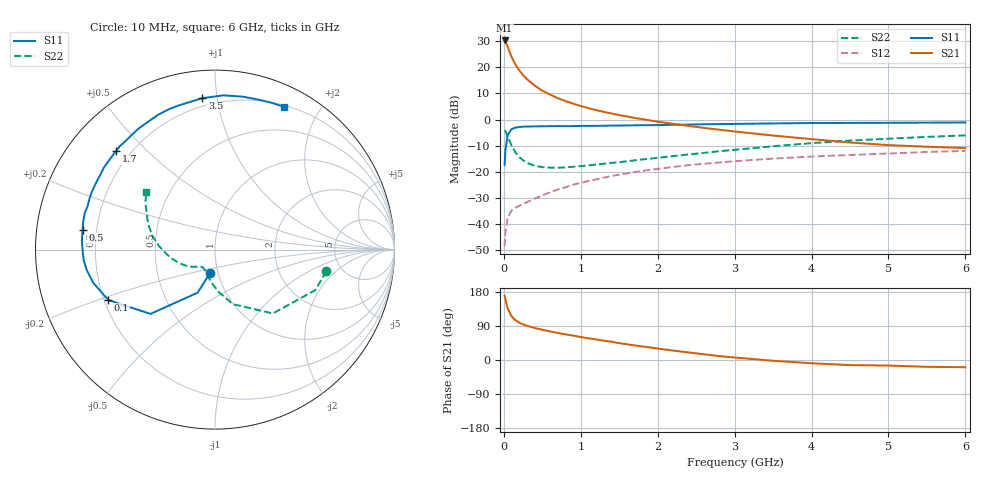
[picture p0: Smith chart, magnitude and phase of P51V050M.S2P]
! SIEMENS Small Signal Semiconductors
! BFP183
! Si NPN RF Bipolar Junction Transistor in SOT143
! VCE = 1 V  IC = 50 mA
! Common Emitter S-Parameters:  March  1996
# GHz  S  MA  R  50
!  f  S11  S21  S12  S22
! GHz  MAG  ANG  MAG  ANG  MAG  ANG  MAG  ANG
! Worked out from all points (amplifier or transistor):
!   36 points, 10 MHz to 6 GHz, reference 50 ohm
!   highest |S21| = 30.3 dB at 10 MHz (marker M1)
!   |S21| within 3 dB of that: start of sweep to 57.36 MHz
!   unconditionally stable (mu >= 1): start of sweep to 34.36 MHz; 150 MHz to end of sweep
!   at 250 MHz: K = 1.32, MAG = 21.3 dB, |S12| = -32.3 dB
!   at 1.4 GHz: K = 1.90, MAG = 6.5 dB, |S12| = -21.6 dB
!   at 6 GHz: K = 1.53, MAG = -3.7 dB, |S12| = -12.0 dB
!   S11 on the Smith chart (normalised r, x): 10 MHz: 0.91, -0.25; 100 MHz: 0.22, -0.21; 500 MHz: 0.15, +0.07; 1.7 GHz: 0.15, +0.40; 3.5 GHz: 0.15, +0.91; 6 GHz: 0.22, +1.57
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0.01  0.1361 -102.5  32.69 169.6  0.0038 64.0  0.6319 -11.0
0.02  0.2584 -111.9  31.52 159.5  0.0069 64.8  0.6033 -21.9
0.05  0.5075 -135.1  24.7 135.9  0.0133 53.1  0.4802 -47.8
0.1  0.6576 -154.7  15.89 115.5  0.0183 41.5  0.3199 -71.8
0.15  0.703 -164.7  11.36 105.1  0.0206 40.7  0.2378 -84.9
0.2  0.7231 -170.8  8.736 98.7  0.0225 42.4  0.193 -94.0
0.25  0.7337 -175.1  7.085 94.0  0.0242 44.3  0.1668 -100.5
0.3  0.7367 -178.6  5.946 90.4  0.0265 46.8  0.1492 -105.7
0.4  0.7434 176.2  4.483 84.5  0.0309 51.0  0.1314 -113.6
0.5  0.7459 171.6  3.582 79.8  0.0356 53.5  0.1235 -119.0
0.6  0.7507 168.0  3.024 75.5  0.0407 56.1  0.1208 -122.5
0.7  0.7542 164.4  2.579 71.5  0.0459 57.8  0.1203 -125.6
0.9  0.754 158.4  2.023 64.4  0.0569 58.6  0.1255 -130.2
1.1  0.7592 151.9  1.661 57.2  0.0673 58.6  0.1334 -134.5
1.3  0.7633 146.4  1.406 50.9  0.0779 57.6  0.1432 -137.9
1.7  0.7784 135.2  1.075 38.5  0.0993 54.4  0.1663 -145.4
2.2  0.797 122.6  0.832 24.9  0.1244 49.0  0.2009 -156.1
2.8  0.8228 108.5  0.642 10.3  0.1515 41.9  0.2488 -168.8
3.5  0.8465 94.8  0.496 -2.0  0.1796 33.8  0.3101 177.0
4.5  0.8659 79.8  0.365 -13.4  0.2107 22.4  0.3974 159.4
5.5  0.8767 69.0  0.303 -18.0  0.2407 12.6  0.468 146.0
6  0.8834 64.2  0.287 -19.1  0.2517 7.3  0.4995 140.0
